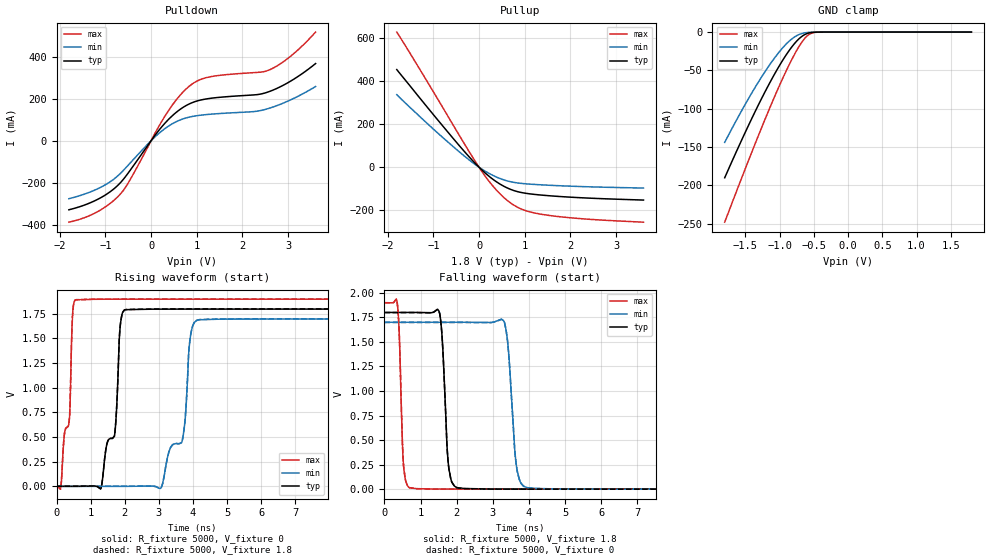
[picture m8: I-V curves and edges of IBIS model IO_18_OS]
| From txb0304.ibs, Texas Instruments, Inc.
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[Model]   IO_18_OS
Model_type  I/O
Vinl=0.595
Vinh=1.235
Enable   Active-High
Vref =   0
Rref =   5000
Cref =   15p
Vmeas =   0.9
| variable   typ   min   max
C_comp   3.79pF   3.50pF   3.98pF
| C_pullup   7.75pF   5.13pF   9.28pF
| C_pulldown   7.88pF   3.20pF   10.76pF
| C_tri-state   3.79pF   3.50pF   3.98pF
[Temperature Range]   40   100   -40
| Ambient temperature   25   85   -40
[Voltage range]   1.8   1.7   1.9
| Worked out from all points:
|   slope of the pulldown table from 0 to 0.27 V, typ, clamps not added: 3.59 ohm
|   slope of the pullup table from 0 to 0.27 V, typ, clamps not added: 5.36 ohm
|   GND clamp passes 1 mA (typ) near -0.56 V on its own axis
|   rising waveform, R_fixture 5000, V_fixture 0: 20-80 % time 393ps typ, 591ps min, 249ps max; typ from 0 V to 1.8 V
|   falling waveform, R_fixture 5000, V_fixture 1.8: 20-80 % time 132ps typ, 178ps min, 91.7ps max; typ from 1.8 V to 0.001 V
|   rising waveform, R_fixture 5000, V_fixture 1.8: 20-80 % time 393ps typ, 591ps min, 249ps max; typ from 0.001 V to 1.8 V
|   falling waveform, R_fixture 5000, V_fixture 0: 20-80 % time 132ps typ, 178ps min, 91.7ps max; typ from 1.8 V to 0 V
[GND Clamp]
| IO_18A
|   Voltage   I(typ)   I(min)   I(max)
-1.8V     -190.1mA   -143.9mA   -248mA
-1.585V   -147.2mA   -107.8mA   -197.9mA
-1.39V    -110mA     -77.2mA    -153.3mA
-1.215V   -78.52mA   -52.06mA   -114.6mA
-1.055V   -52.01mA   -31.68mA   -80.7mA
-910mV    -30.68mA   -16.27mA   -52.03mA
-785mV    -15.38mA   -6.585mA   -29.67mA
-675mV    -5.707mA   -1.924mA   -13.21mA
-585mV    -1.52mA    -502.6uA   -4.193mA
-515mV    -365.4uA   -143.1uA   -1.022mA
-410mV    -26.79uA   -12.71uA   -53.57uA
1.8V      537.4pA    18.6nA     37.53pA
[Pulldown]
| IO_18A
|   Voltage   I(typ)   I(min)   I(max)
-1.8V     -328.4mA   -275.8mA   -387.5mA
-1.175V   -279.5mA   -229.1mA   -338mA
-675mV    -200.4mA   -156.1mA   -254.1mA
-455mV    -139.7mA   -105.5mA   -183.7mA
275mV     76.47mA    53.15mA    107mA
575mV     139.1mA    92.84mA    200.7mA
860mV     177.3mA    113.4mA    263.4mA
1.29V     201.2mA    125.8mA    303.8mA
2.25V     217.7mA    138.5mA    323.7mA
2.59V     234mA      154.6mA    336.7mA
3.06V     284.1mA    194.8mA    402.7mA
3.6V      366.8mA    257.6mA    516.4mA
[Pullup]
| IO_18A
|   Voltage   I(typ)   I(min)   I(max)
-1.8V     451.7mA    335.5mA    625.2mA
-765mV    183.6mA    132.1mA    266.1mA
-315mV    71.4mA     50.6mA     106.4mA
5mV       -1.045mA   -722.9uA   -1.605mA
330mV     -59.85mA   -40.6mA    -93.7mA
490mV     -81.85mA   -54.78mA   -129.7mA
645mV     -98.49mA   -64.88mA   -158.2mA
805mV     -110.8mA   -71.67mA   -180.9mA
975mV     -119mA     -75.88mA   -197.6mA
1.435V    -130.3mA   -82.41mA   -220.1mA
2.3V      -142mA     -89.98mA   -239.2mA
3.6V      -152.1mA   -96.51mA   -254.4mA
[Ramp]
| IO_18A
| variable   typ   min   max
dV/dt_r   1.10/3.99E-10   1.03/6.03E-10   1.16/2.54E-10
dV/dt_f   1.10/1.47E-10   1.04/1.97E-10   1.16/9.62E-11
R_load = 5000
[Rising Waveform]
| IO_18A
R_fixture =   5000
C_fixture =   0
L_fixture =   0
V_fixture =   0
V_fixture_min = 0
V_fixture_max = 0
|   Time   V(typ)   V(min)   V(max)
0s        1.256nV    7.922nV    126.5pV
369ps     -3.382uV   7.885nV    655.8mV
467ps     -6.911uV   2.365nV    1.717V
579ps     -4.863uV   -7.604nV   1.893V
1.307ns   -14.75mV   281nV      1.898V
2.049ns   1.793V     5.618uV    1.899V
3.673ns   1.798V     443.6mV    1.899V
3.925ns   1.798V     1.512V     1.899V
4.205ns   1.798V     1.69V      1.899V
66.81ns   1.798V     1.698V     1.899V
[Falling Waveform]
| IO_18A
R_fixture =   5000
C_fixture =   0
L_fixture =   0
V_fixture =   1.8
V_fixture_min = 1.7
V_fixture_max = 1.9
|   Time   V(typ)   V(min)   V(max)
0s        1.8V       1.7V       1.9V
341ps     1.8V       1.7V       1.925V
887ps     1.8V       1.7V       5.442mV
1.531ns   1.788V     1.7V       1.193mV
1.783ns   213.1mV    1.7V       1.049mV
2.231ns   6.4mV      1.7V       954.2uV
3.323ns   1.299mV    1.698V     907.3uV
3.673ns   1.232mV    194.7mV    904.2uV
4.205ns   1.194mV    7.603mV    901.7uV
66.81ns   1.163mV    1.533mV    897.7uV
[Rising Waveform]
| IO_18A
R_fixture =   5000
C_fixture =   0
L_fixture =   0
V_fixture =   1.8
V_fixture_min = 1.7
V_fixture_max = 1.9
|   Time   V(typ)   V(min)   V(max)
0s        1.163mV    1.533mV    897.7uV
369ps     1.159mV    1.533mV    657.3mV
467ps     1.156mV    1.533mV    1.719V
579ps     1.158mV    1.533mV    1.894V
1.307ns   -13.59mV   1.534mV    1.899V
2.049ns   1.794V     1.539mV    1.9V
3.673ns   1.8V       445.9mV    1.9V
3.925ns   1.8V       1.516V     1.9V
4.205ns   1.8V       1.693V     1.9V
66.81ns   1.8V       1.7V       1.9V
[Falling Waveform]
| IO_18A
R_fixture =   5000
C_fixture =   0
L_fixture =   0
V_fixture =   0
V_fixture_min = 0
V_fixture_max = 0
|   Time   V(typ)   V(min)   V(max)
0s        1.798V     1.698V     1.899V
341ps     1.798V     1.698V     1.924V
887ps     1.798V     1.698V     4.534mV
1.531ns   1.786V     1.698V     294.2uV
1.783ns   210.4mV    1.698V     150.7uV
2.231ns   5.215mV    1.698V     56.34uV
3.323ns   135.6uV    1.695V     9.605uV
3.673ns   69.28uV    190.5mV    6.485uV
4.205ns   31.5uV     6.019mV    4.042uV
66.81ns   11.84nV    80.07nV    24.22nV
